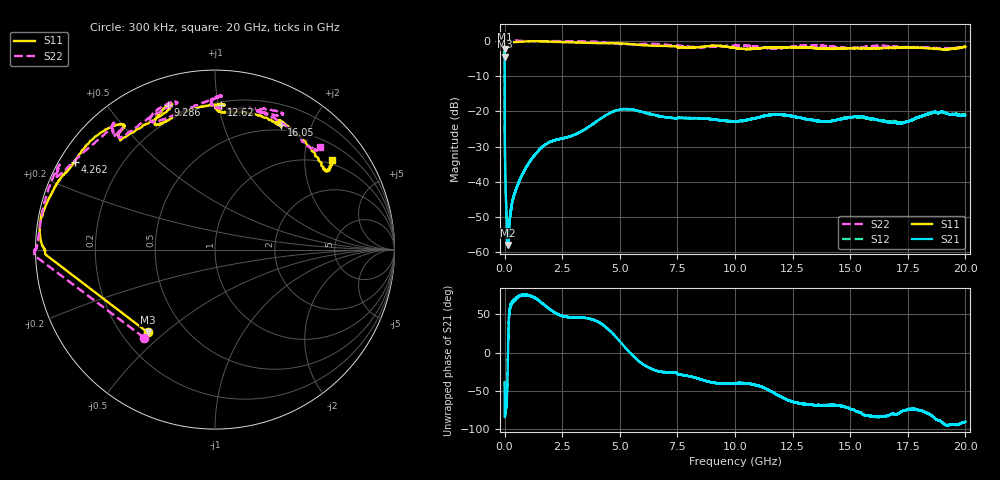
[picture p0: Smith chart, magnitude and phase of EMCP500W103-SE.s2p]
!EMCP500W103
!Johanson Technology Inc.
!www.johansontechnology.com
!Test Board Conditions:
!Substrate Type  RO4350B
!Substrate Thickness  10 mil
!Substrate Dk  3.66
!TL Type: GCPW
!TL Trace Width  20 mil
!TL Gap  10 mil
!PART MODE SINGLE ENDED (AKA BYPASS)
!DUT TOPOLOGY	SERIES-SHUNT
# MHz S  dB  R 50
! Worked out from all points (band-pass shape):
!   20001 points, 300 kHz to 20 GHz, reference 50 ohm
!   highest |S21| = -2.39 dB at 300 kHz (marker M1); lowest = -57.9 dB at 148.3 MHz (marker M2)
!   |S21| within 3 dB of the highest: start of sweep to 638.7 kHz
!   lowest |S11| = -4.5 dB at 300 kHz (marker M3), VSWR 3.93, Z = 15.4 - j21.9 ohm
!   |S11| at or under -10 dB: nowhere
!   |S22| runs from -4.0 to 0.1 dB; largest |S21 - S12| = 0.0051
!   S11 on the Smith chart (normalised r, x): 300 kHz: 0.31, -0.44; 4.262 GHz: 0.04, +0.29; 9.286 GHz: 0.13, +0.72; 12.62 GHz: 0.22, +1.02; 16.05 GHz: 0.43, +1.57; 20 GHz: 0.89, +2.70
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0.3  -4.52 -129.1  -2.39 -38.9  -2.39 -39.0  -4.01 -128.8
101.298  -0.47 -179.8  -51.99 -57.8  -52.29 -60.7  0.05 -179.7
148.298  -0.46 -179.8  -57.90 0.4  -57.49 3.7  0.06 -179.8
534.292  -0.36 178.9  -41.53 71.5  -41.43 72.5  0.00 -179.9
1252.281  -0.12 171.2  -32.85 72.5  -32.85 72.4  -0.13 175.0
2323.265  -0.35 160.4  -27.94 49.7  -27.99 49.9  -0.10 153.7
3334.25  -0.53 153.5  -25.69 45.8  -25.72 45.6  -0.17 153.7
4262.236  -0.70 148.0  -21.66 36.5  -21.71 36.8  -0.44 152.6
6667.2  -1.43 127.7  -21.29 -24.3  -21.36 -23.9  -0.93 129.3
7452.188  -1.59 130.2  -21.99 -26.7  -21.95 -26.5  -1.41 131.2
8258.176  -1.91 113.5  -21.93 -32.9  -21.97 -32.8  -1.80 129.3
9286.161  -1.45 108.1  -22.50 -40.4  -22.46 -40.9  -1.59 108.7
10000.15  -2.05 115.2  -22.86 -40.1  -22.99 -40.3  -1.41 105.0
11252.13  -2.02 99.0  -21.40 -46.0  -21.26 -45.9  -1.93 116.5
12622.11  -1.87 87.5  -21.56 -65.2  -21.61 -65.2  -1.64 92.5
13334.1  -2.02 89.8  -22.45 -68.2  -22.50 -68.1  -1.34 87.7
14708.08  -2.18 79.7  -22.07 -70.7  -21.91 -70.7  -2.02 89.7
16046.06  -2.10 62.1  -22.20 -83.6  -22.29 -82.4  -1.46 66.5
16667.05  -2.05 62.8  -23.15 -82.3  -22.94 -81.3  -1.56 63.9
17882.03  -1.97 60.0  -21.88 -75.0  -21.92 -75.8  -1.89 71.9
19080.01  -2.44 37.0  -20.32 -93.6  -20.38 -91.8  -2.23 49.3
20000  -1.72 37.3  -21.15 -90.7  -20.77 -91.2  -1.74 44.4
